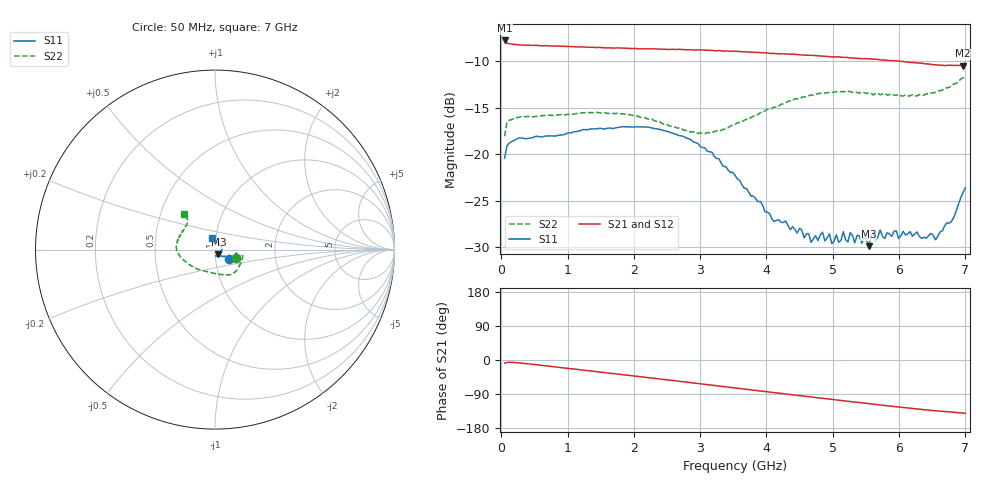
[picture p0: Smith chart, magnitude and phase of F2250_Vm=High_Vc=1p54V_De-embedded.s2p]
! Integrated Device Technology
! Corporate Headquarters
! 6024 Silver Creek Valley Road
! San Jose, CA 95138  USA
! Phone:  1-408-284-8200
! Toll Free:  1-800-223-1366
! Webpage:  http://www.idt.com/
! Timing and RF Division
! 515 Groton Road, Suite 102
! Westford, MA 01886-6024
! Device:  F2250
! Description: Voltage Variable RF Attenuator
! Frequency:  50.0 -  6000.00 MHz
! Package:  3x3 mm Thin QFN Plastic Package: 16 pin
! Ports:  2 RF, 3 DC
!  Pin  1  = GND
!  Pin  2  = NC
!  Pin  3  = RF1  = Port 1
!  Pin  4  = NC
!  Pin  5  = GND
!  Pin  6  = GND
!  Pin  7  = GND
!  Pin  8  = GND
!  Pin  9  = NC
!  Pin 10  = RF2  = Port 2
!  Pin 11  = NC
!  Pin 12  = GND
!  Pin 13  = GND
!  Pin 14  = VCNTRL
!  Pin 15  = VDD
!  Pin 16  = VMODE
! Vcntrl:  1.540 Volts
! Vmode:  +3.300 Volts
! Vdd:  +3.30  Volts
! Current:  1.329 mA
! Data:  The device was measured on a the F2250 evaluation board which has
!  individual transmission lines to the RF pins.  Data was collected
!  using a calibrated network analyzer.  The evaluation board was
!  de-embedded using a TRL calibration technique.
!  The reference plane is the edge of the package pin.
! Misc:  SN 10
!  Action Tracker AT0258
! Date Measured:  2014-11-26
! Date:  2015-10-15  MJV
! Note:
!  Integrated Device Technology supplies this data as a sample of measured
!  data at the package pin for this product.  Your particular data for this
!  product may vary.
!  Data was taken at 25 degrees C.
!  Integrated Device Technology reserves the right to change this data at anytime.
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# GHz S dB R 50
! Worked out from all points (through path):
!   201 points, 50 MHz to 7 GHz, reference 50 ohm
!   highest |S21| = -7.75 dB at 50 MHz (marker M1); lowest = -10.5 dB at 6.965 GHz (marker M2)
!   group delay of S21, straight-line fit = 56.2 ps
!   lowest |S11| = -29.9 dB at 5.54 GHz (marker M3), VSWR 1.07, Z = 51.9 - j2.65 ohm
!   |S11| at or under -10 dB: start of sweep to end of sweep
!   |S22| runs from -18.1 to -11.6 dB; largest |S21 - S12| = 0.002
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0.05  -20.41 -35.1  -7.75 -8.5  -7.75 -8.5  -18.05 -23.0
0.08475  -19.11 -17.5  -8.04 -6.5  -8.00 -6.4  -16.58 -12.7
0.2585  -18.26 -9.9  -8.21 -7.4  -8.21 -7.4  -16.02 -12.9
1.2315  -17.35 -22.6  -8.45 -26.7  -8.47 -26.7  -15.53 -42.4
2.37825  -17.31 -23.7  -8.69 -49.8  -8.70 -49.8  -16.46 -70.8
2.969  -18.86 -23.3  -8.77 -62.1  -8.79 -62.1  -17.76 -98.0
3.525  -22.26 -31.0  -8.91 -73.8  -8.92 -73.8  -16.79 -131.4
4.11575  -27.24 -54.2  -9.15 -86.1  -9.15 -86.1  -14.92 -158.1
4.7065  -29.11 -78.3  -9.36 -98.3  -9.37 -98.3  -13.64 -175.1
4.8455  -28.38 -73.9  -9.45 -101.1  -9.44 -101.1  -13.43 -178.2
5.08875  -29.47 -71.1  -9.52 -106.2  -9.53 -106.2  -13.32 175.7
5.15825  -28.33 -71.2  -9.57 -107.5  -9.56 -107.6  -13.24 174.3
5.22775  -29.45 -71.2  -9.59 -109.0  -9.59 -109.0  -13.24 172.4
5.5405  -29.89 -52.8  -9.74 -115.2  -9.72 -115.3  -13.38 164.3
5.61  -28.37 -47.0  -9.76 -116.6  -9.76 -116.6  -13.61 163.0
5.64475  -29.30 -45.1  -9.79 -117.3  -9.79 -117.4  -13.48 161.0
5.71425  -28.14 -42.8  -9.84 -118.6  -9.84 -118.7  -13.60 160.2
5.85325  -28.55 -32.7  -9.93 -121.3  -9.90 -121.5  -13.59 155.7
6.54825  -29.20 40.6  -10.37 -133.9  -10.39 -134.0  -13.35 135.3
6.7915  -27.21 77.2  -10.43 -137.4  -10.44 -137.5  -12.61 131.6
6.96525  -24.09 103.8  -10.46 -140.1  -10.46 -140.2  -11.79 132.2
7  -23.60 106.7  -10.43 -140.6  -10.43 -140.8  -11.60 131.5
